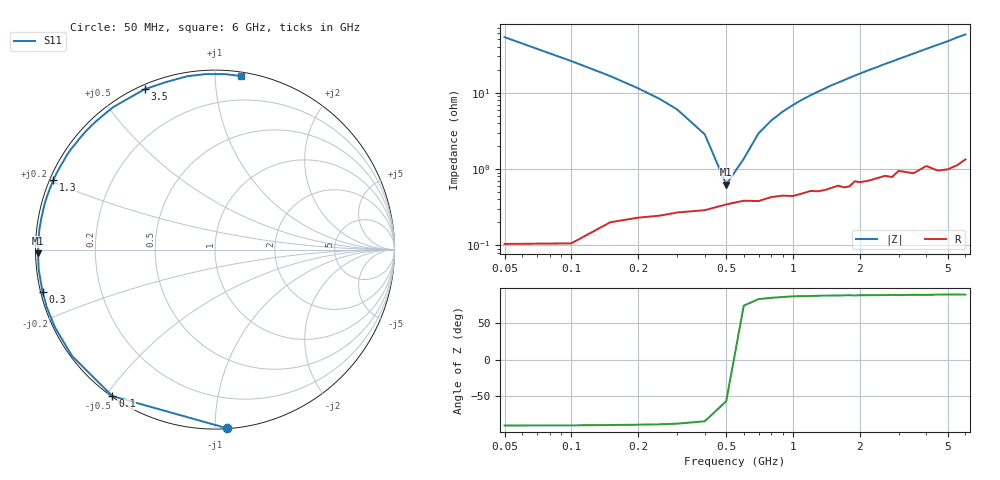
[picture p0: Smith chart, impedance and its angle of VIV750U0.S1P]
! Infineon Technologies  Discrete & RF Semiconductors
! BB 804
! Si Tuning Diode in SOT23
! VR = 0.75 V
! S-Parameters:  July  1999
# GHz  S  MA  R  50
!  f  S11
! GHz  MAG  ANG
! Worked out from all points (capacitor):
!   34 points, 50 MHz to 6 GHz, reference 50 ohm
!   read as one part to ground: C = 59 pF near 50 MHz
!   lowest |Z| = 626 mohm at 500 MHz (marker M1)
!   series resonance near 528.6 MHz, so ESL is about 1.5 nH
!   S11 on the Smith chart (normalised r, x): 50 MHz: 0.00, -1.07; 100 MHz: 0.00, -0.52; 300 MHz: 0.01, -0.12; 1.3 GHz: 0.01, +0.21; 3.5 GHz: 0.02, +0.65; 6 GHz: 0.03, +1.16
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0.05  0.9981 -86.1
0.1  0.9967 -125.0
0.15  0.9928 -143.4
0.2  0.9913 -154.2
0.25  0.9905 -161.1
0.3  0.9895 -166.2
0.4  0.9886 -173.5
0.5  0.9864 -178.8
0.6  0.9848 177.0
0.7  0.9849 173.3
0.8  0.9831 170.1
1  0.9828 164.3
1.3  0.9806 156.6
1.5  0.9788 151.7
1.6  0.9777 149.6
1.8  0.9787 145.1
2  0.9764 140.9
2.2  0.9759 136.7
2.4  0.9748 133.0
2.6  0.9738 129.0
2.8  0.9754 125.6
3  0.9715 121.9
3.5  0.9756 113.7
4  0.9725 106.0
4.5  0.9781 99.1
5  0.9794 93.0
5.5  0.9792 86.5
6  0.9775 81.4
